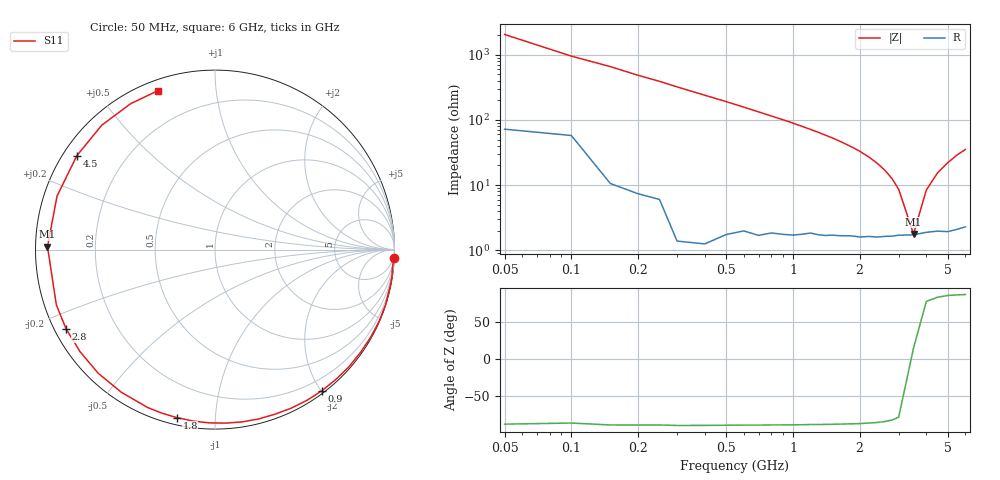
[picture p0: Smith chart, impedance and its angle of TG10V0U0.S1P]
! SIEMENS Discrete & RF Semiconductors
! BAT64
! Si Schottky Diode in SOT23
! VR = 10 V
! S-Parameters:  February  1997
# GHz  S  MA  R  50
!  f  S11
! GHz  MAG  ANG
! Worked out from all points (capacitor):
!   34 points, 50 MHz to 6 GHz, reference 50 ohm
!   read as one part to ground: C = 1.61 pF near 50 MHz
!   lowest |Z| = 1.78 ohm at 3.5 GHz (marker M1)
!   series resonance near 3.475 GHz, so ESL is about 1.3 nH
!   S11 on the Smith chart (normalised r, x): 50 MHz: 1, -41; 900 MHz: 0.04, -2.01; 1.8 GHz: 0.03, -0.80; 2.8 GHz: 0.03, -0.25; 4.5 GHz: 0.04, +0.31; 6 GHz: 0.05, +0.70
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0.05  0.9983 -2.8
0.2  0.9969 -11.8
0.3  0.9987 -17.7
0.4  0.9979 -23.6
0.5  0.9955 -29.4
0.6  0.9927 -35.3
0.7  0.9916 -41.3
0.8  0.9883 -47.1
0.9  0.9862 -52.8
1  0.9838 -58.5
1.1  0.9803 -64.3
1.3  0.9744 -75.5
1.4  0.9719 -81.1
1.6  0.9659 -92.0
1.7  0.963 -97.4
1.8  0.9601 -102.8
2  0.9565 -113.1
2.2  0.9507 -123.3
2.4  0.9477 -133.3
2.6  0.943 -142.8
2.8  0.9398 -152.0
3  0.9359 -160.8
3.5  0.9334 179.0
4  0.9292 161.3
4.5  0.9307 145.8
5  0.9373 132.3
5.5  0.939 120.0
6  0.9406 109.8
